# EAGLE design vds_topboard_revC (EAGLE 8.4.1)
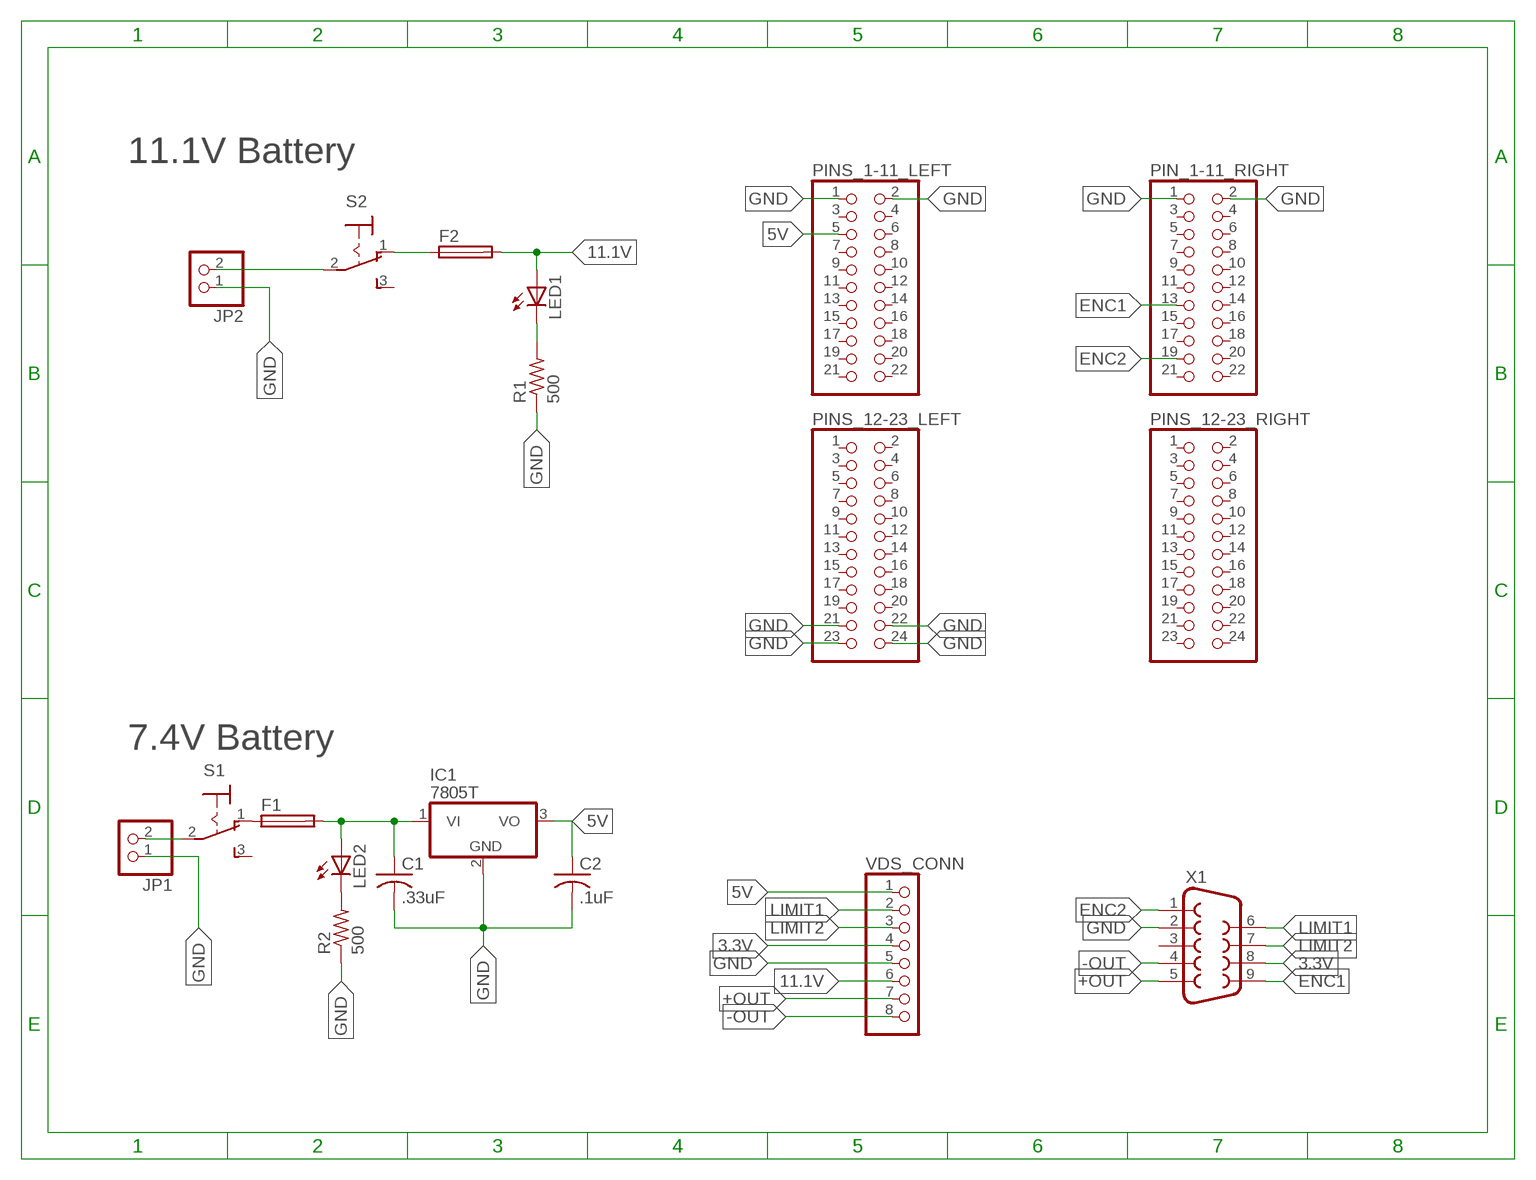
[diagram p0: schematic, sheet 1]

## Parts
C1  .33uF  C-US025-030X050  [C025-030X050]
C2  .1uF  C-US025-030X050  [C025-030X050]
F1  SH22,5  [SH22,5]
F2  SH22,5  [SH22,5]
IC1  7805T  [TO220H]
JP1  PINHD-1X2  [1X02]
JP2  PINHD-1X2  [1X02]
LED1  LED5MM  [LED5MM]
LED2  LED5MM  [LED5MM]
PIN_1-11_RIGHT  PINHD-2X11  [2X11]
PINS_1-11_LEFT  PINHD-2X11  [2X11]
PINS_12-23_LEFT  PINHD-2X12  [2X12]
PINS_12-23_RIGHT  PINHD-2X12  [2X12]
R1  500  R-US_0204/5  [0204/5]
R2  500  R-US_0204/5  [0204/5]
S1  320-916  [320-916]
S2  320-916  [320-916]
VDS_CONN  PINHD-1X8  [1X08]
X1  F09VP  [F09VP]

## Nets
3.3V: VDS_CONN.4 X1.8
5V: C2.1 IC1.3(VO) PINS_1-11_LEFT.5 VDS_CONN.1
7.4VO: C1.1 F1.2 IC1.1(VI) LED2.A
11.1V: F2.2 LED1.A VDS_CONN.6
+OUT: VDS_CONN.7 X1.5
-OUT: VDS_CONN.8 X1.4
ENC1: PIN_1-11_RIGHT.13 X1.9
ENC2: PIN_1-11_RIGHT.19 X1.1
GND: C1.2 C2.2 IC1.2(GND) JP1.1 JP2.1 PIN_1-11_RIGHT.1 PIN_1-11_RIGHT.2 PINS_1-11_LEFT.1 PINS_1-11_LEFT.2 PINS_12-23_LEFT.21 PINS_12-23_LEFT.22 PINS_12-23_LEFT.23 PINS_12-23_LEFT.24 R1.1 R2.1 VDS_CONN.5 X1.2
LIMIT1: VDS_CONN.2 X1.6
LIMIT2: VDS_CONN.3 X1.7
N$1: JP1.2 S1.2(P)
N$2: JP2.2 S2.2(P)
N$4: F2.1 S2.1(O)
N$5: LED1.K(C) R1.2
N$6: LED2.K(C) R2.2
N$7: F1.1 S1.1(O)
Unconnected: PIN_1-11_RIGHT.3 PIN_1-11_RIGHT.4 PIN_1-11_RIGHT.5 PIN_1-11_RIGHT.6 PIN_1-11_RIGHT.7 PIN_1-11_RIGHT.8 PIN_1-11_RIGHT.9 PIN_1-11_RIGHT.10 PIN_1-11_RIGHT.11 PIN_1-11_RIGHT.12 PIN_1-11_RIGHT.14 PIN_1-11_RIGHT.15 PIN_1-11_RIGHT.16 PIN_1-11_RIGHT.17 PIN_1-11_RIGHT.18 PIN_1-11_RIGHT.20 PIN_1-11_RIGHT.21 PIN_1-11_RIGHT.22 PINS_1-11_LEFT.3 PINS_1-11_LEFT.4 PINS_1-11_LEFT.6 PINS_1-11_LEFT.7 PINS_1-11_LEFT.8 PINS_1-11_LEFT.9 PINS_1-11_LEFT.10 PINS_1-11_LEFT.11 PINS_1-11_LEFT.12 PINS_1-11_LEFT.13 PINS_1-11_LEFT.14 PINS_1-11_LEFT.15 PINS_1-11_LEFT.16 PINS_1-11_LEFT.17 PINS_1-11_LEFT.18 PINS_1-11_LEFT.19 PINS_1-11_LEFT.20 PINS_1-11_LEFT.21 PINS_1-11_LEFT.22 PINS_12-23_LEFT.1 PINS_12-23_LEFT.2 PINS_12-23_LEFT.3 PINS_12-23_LEFT.4 PINS_12-23_LEFT.5 PINS_12-23_LEFT.6 PINS_12-23_LEFT.7 PINS_12-23_LEFT.8 PINS_12-23_LEFT.9 PINS_12-23_LEFT.10 PINS_12-23_LEFT.11 PINS_12-23_LEFT.12 PINS_12-23_LEFT.13 PINS_12-23_LEFT.14 PINS_12-23_LEFT.15 PINS_12-23_LEFT.16 PINS_12-23_LEFT.17 PINS_12-23_LEFT.18 PINS_12-23_LEFT.19 PINS_12-23_LEFT.20 PINS_12-23_RIGHT.1 PINS_12-23_RIGHT.2 PINS_12-23_RIGHT.3 PINS_12-23_RIGHT.4 PINS_12-23_RIGHT.5 PINS_12-23_RIGHT.6 PINS_12-23_RIGHT.7 PINS_12-23_RIGHT.8 PINS_12-23_RIGHT.9 PINS_12-23_RIGHT.10 PINS_12-23_RIGHT.11 PINS_12-23_RIGHT.12 PINS_12-23_RIGHT.13 PINS_12-23_RIGHT.14 PINS_12-23_RIGHT.15 PINS_12-23_RIGHT.16 PINS_12-23_RIGHT.17 PINS_12-23_RIGHT.18 PINS_12-23_RIGHT.19 PINS_12-23_RIGHT.20 PINS_12-23_RIGHT.21 PINS_12-23_RIGHT.22 PINS_12-23_RIGHT.23 PINS_12-23_RIGHT.24 S1.3(S) S2.3(S) X1.3

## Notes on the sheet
- 11.1V Battery
- 7.4V Battery

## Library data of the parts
C1 C2 = adafruit:C-US: CAPACITOR, American symbol
F1 F2 = fuse:SH22,5: FUSE HOLDER; MF: SCHURTER; MPN: 0031.8201; OC_FARNELL: 1162740; OC_NEWARK: 96F8317
IC1 = linear:78*: Positive VOLTAGE REGULATOR Source: http://cache.national.com/ds/LM/LM78L05.pdf http://www.fairchildsemi.com/ds/LM/LM7805.pdf
JP1 JP2 = pinhead:PINHD-1X2: PIN HEADER
LED1 LED2 = adafruit:LED: LED
PIN_1-11_RIGHT PINS_1-11_LEFT = pinhead:PINHD-2X11: PIN HEADER
PINS_12-23_LEFT PINS_12-23_RIGHT = pinhead:PINHD-2X12: PIN HEADER
R1 R2 = adafruit:R-US_: RESISTOR, American symbol
S1 S2 = switch:320-916: TOGGLE SWITCH distributor RS Components
VDS_CONN = pinhead:PINHD-1X8: PIN HEADER
X1 = con-subd:F09: SUB-D; OC_FARNELL: unknown; OC_NEWARK: unknown

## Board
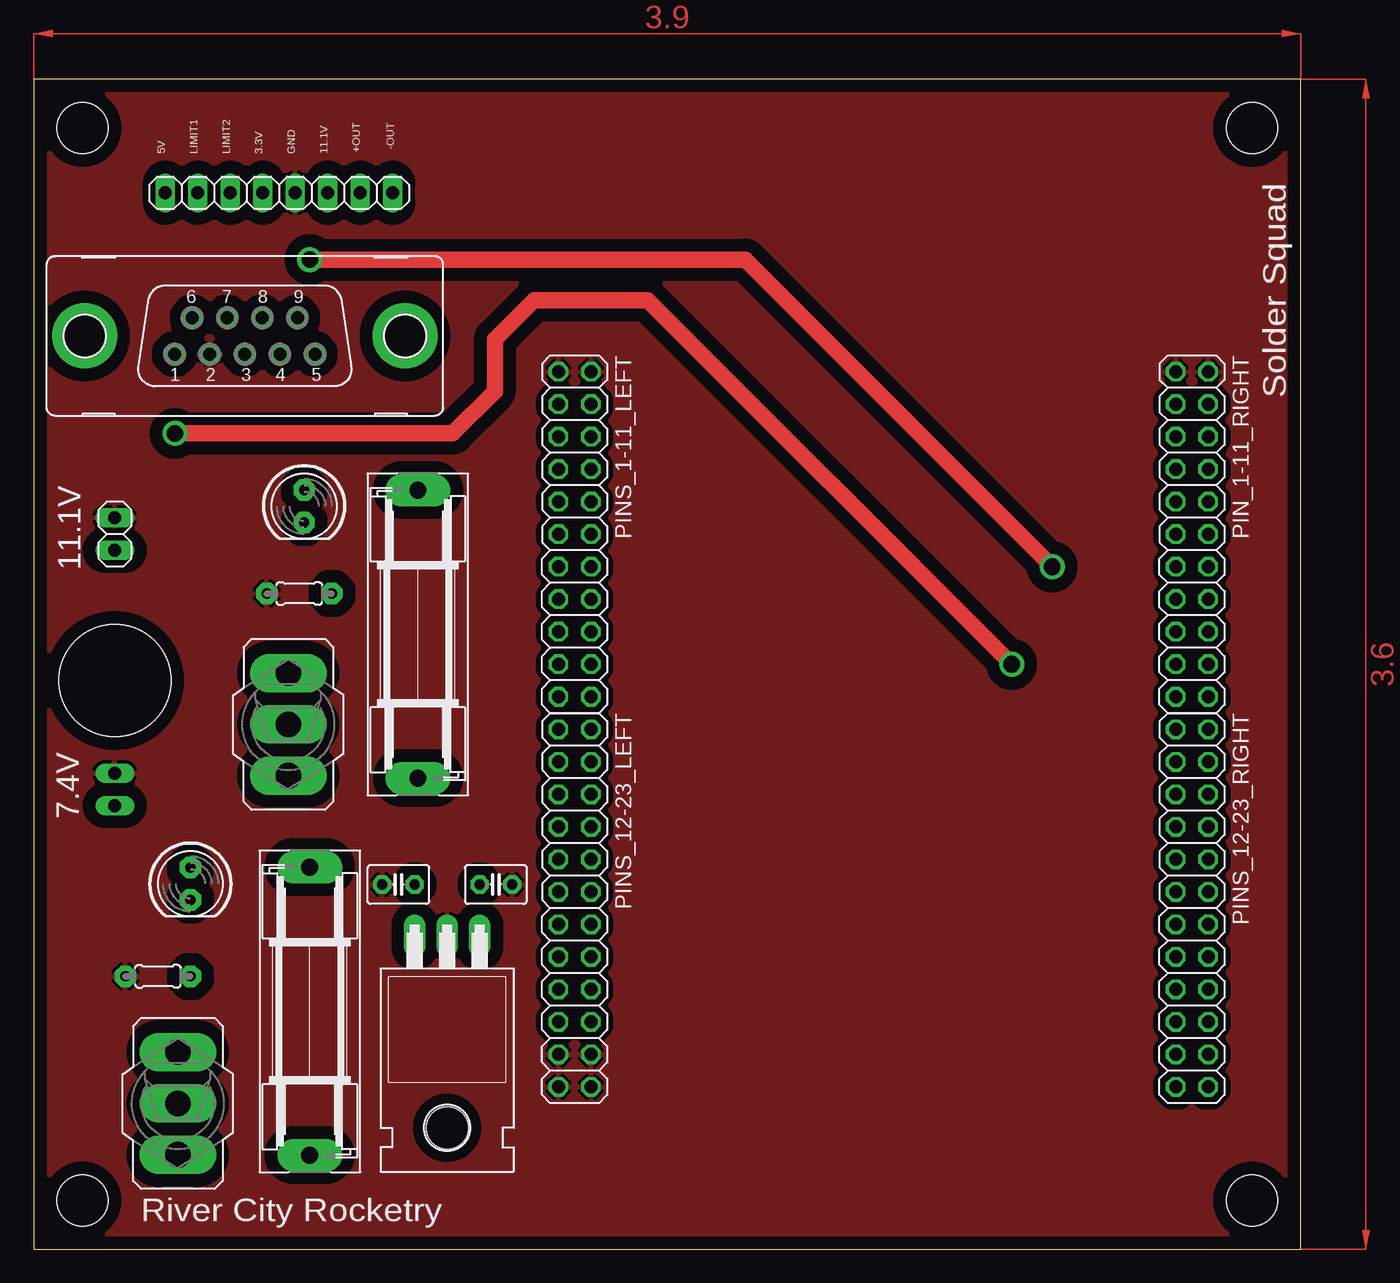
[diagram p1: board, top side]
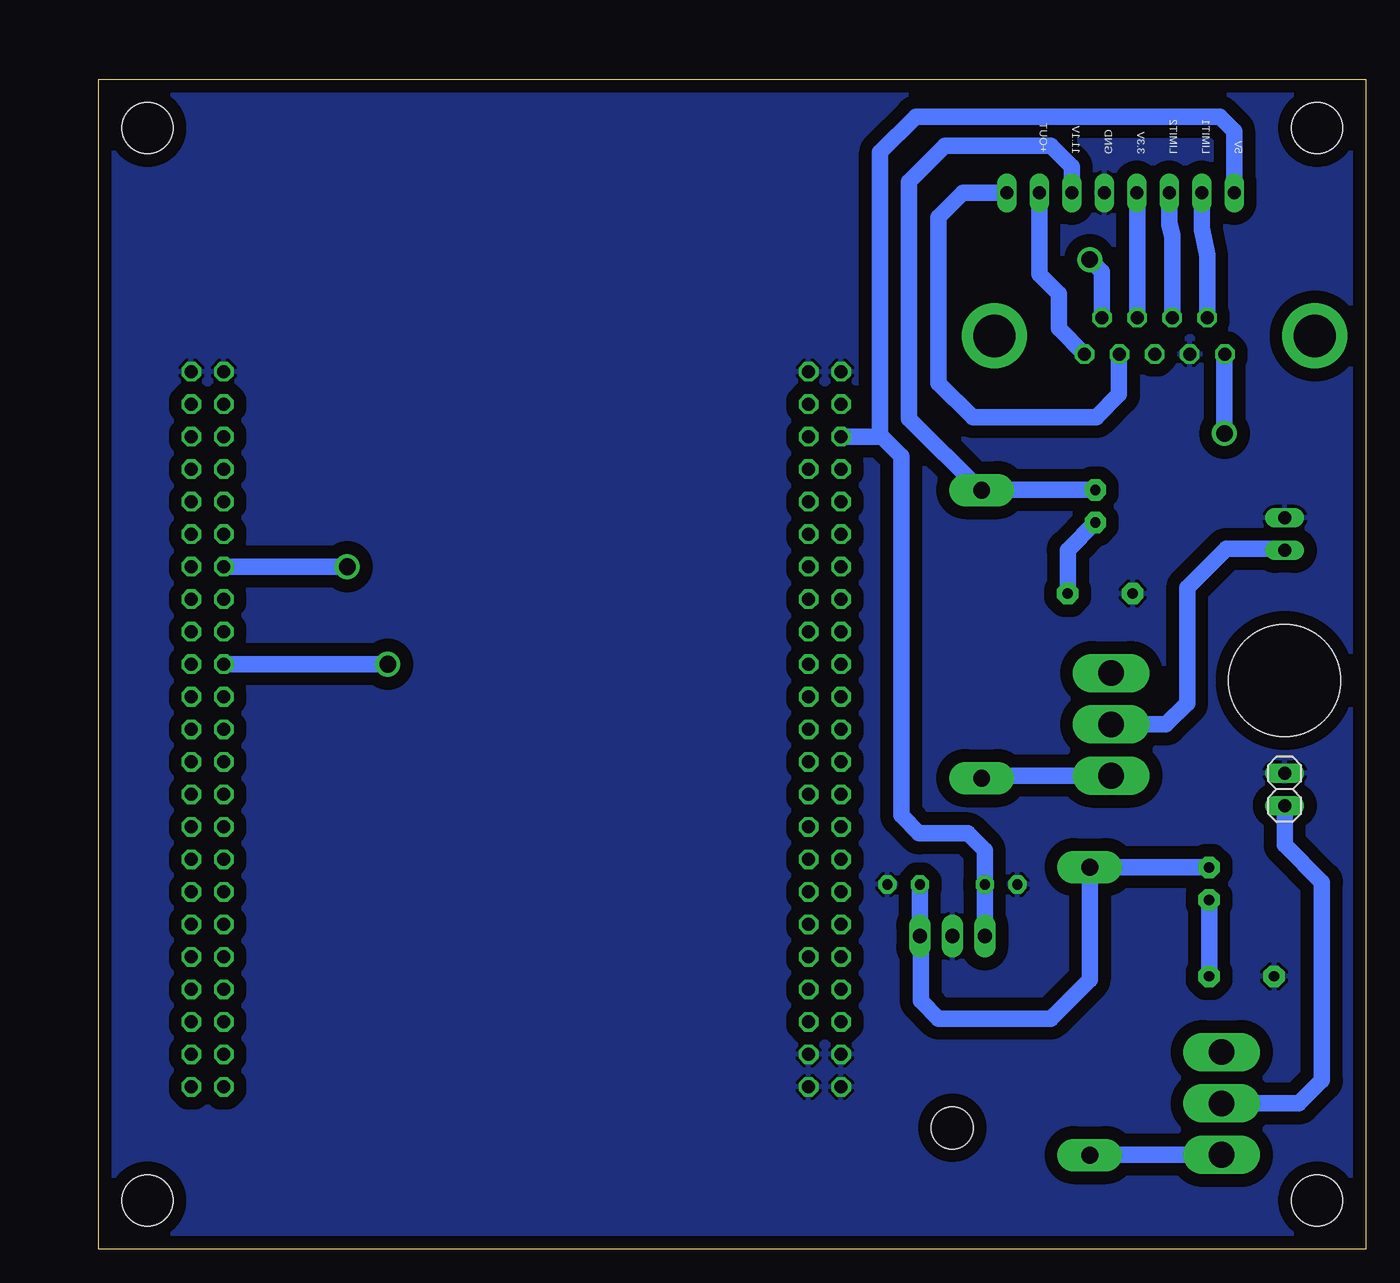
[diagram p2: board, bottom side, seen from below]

Size 99.06 x 91.44 mm. Coordinates in mm from the lower left corner, seen from the top.
Outline: 0,0 99.06,0 99.06,91.44 0,91.44 0,0
Copper layers (1*16): Top 0.035mm / dielectric 1.5mm / Bottom 0.035mm
Design rules "default *": minimum track width 10mil, minimum drill 24mil, track to track 1mm, track to pad 1mm, pad to pad 1mm, via to via 1mm, smd to smd 1mm, copper to edge 40mil, drill to drill 8mil, minimum pad ring 10mil, minimum via ring 8mil, stop-mask expansion 4mil, vias tented up to drill 0mil, thermal gap 10mil
Holes 4 mm at 3.81,3.81 3.81,87.63 95.25,87.63 95.25,3.81
Holes 8.76 mm at 6.35,44.45

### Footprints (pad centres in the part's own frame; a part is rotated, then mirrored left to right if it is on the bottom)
C025-030X050 = drill 0.813 pad 1.422 octagon: 1 -1.27,0; 2 1.27,0
SH22,5 = drill 1.321 pad 2.54 long: 1 -11.252,0; 2 11.252,0
TO220H = drill 1.118 long: 1 -2.54,-10.16; 2 0,-10.16; 3 2.54,-10.16 | hole 3.302: 0,4.826
1X02 = drill 1.016 long: 1 -1.27,0; 2 1.27,0
LED5MM = drill 0.813 pad 1.676 octagon: A -1.27,0; K 1.27,0
2X11 = drill 1.016 octagon: 1 -12.7,-1.27; 2 -12.7,1.27; 3 -10.16,-1.27; 4 -10.16,1.27; 5 -7.62,-1.27; 6 -7.62,1.27; 7 -5.08,-1.27; 8 -5.08,1.27; 9 -2.54,-1.27; 10 -2.54,1.27; 11 0,-1.27; 12 0,1.27; 13 2.54,-1.27; 14 2.54,1.27; 15 5.08,-1.27; 16 5.08,1.27; 17 7.62,-1.27; 18 7.62,1.27; 19 10.16,-1.27; 20 10.16,1.27; 21 12.7,-1.27; 22 12.7,1.27
2X12 = drill 1.016 octagon: 1 -13.97,-1.27; 2 -13.97,1.27; 3 -11.43,-1.27; 4 -11.43,1.27; 5 -8.89,-1.27; 6 -8.89,1.27; 7 -6.35,-1.27; 8 -6.35,1.27; 9 -3.81,-1.27; 10 -3.81,1.27; 11 -1.27,-1.27; 12 -1.27,1.27; 13 1.27,-1.27; 14 1.27,1.27; 15 3.81,-1.27; 16 3.81,1.27; 17 6.35,-1.27; 18 6.35,1.27; 19 8.89,-1.27; 20 8.89,1.27; 21 11.43,-1.27; 22 11.43,1.27; 23 13.97,-1.27; 24 13.97,1.27
0204/5 = drill 0.813 pad 1.676 octagon: 1 -2.54,0; 2 2.54,0
320-916 = drill 2.007 long: 1 0,4.013; 2 0,0; 3 0,-4.013
1X08 = drill 1.016 long: 1 -8.89,0; 2 -6.35,0; 3 -3.81,0; 4 -1.27,0; 5 1.27,0; 6 3.81,0; 7 6.35,0; 8 8.89,0
F09VP = drill 1.016 octagon: 1 5.486,1.422; 2 2.743,1.422; 3 0,1.422; 4 -2.743,1.422; 5 -5.486,1.422; 6 4.115,-1.422; 7 1.372,-1.422; 8 -1.372,-1.422; 9 -4.115,-1.422 | drill 3.302 pad 5.08: G1 -12.522,0; G2 12.522,0

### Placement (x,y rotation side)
C1  36.13,28.51 0 top
C2  28.51,28.51 180 top
F1  21.59,18.61 90 top
F2  30.04,48.07 90 top
IC1  32.32,14.32 180 top
JP1  6.35,35.94 270 bottom
JP2  6.35,55.88 270 top
LED1  21.15,58.07 270 top
LED2  12.26,28.57 270 top
PIN_1-11_RIGHT  90.55,55.88 270 top
PINS_1-11_LEFT  42.29,55.88 270 top
PINS_12-23_LEFT  42.29,26.67 270 top
PINS_12-23_RIGHT  90.55,26.67 270 top
R1  20.76,51.24 0 top
R2  9.72,21.34 0 top
S1  11.27,11.4 180 top
S2  19.91,41.02 180 top
VDS_CONN  19.18,82.55 0 top
X1  16.51,71.37 180 top

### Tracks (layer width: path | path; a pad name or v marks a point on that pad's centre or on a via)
3.3V
  Bottom 1.27: X1.8 17.88,82.53 VDS_CONN.4
5V
  Bottom 1.27: IC1.3 C2.1 29.78,31.18 31.11,32.51 34.92,32.51 36.32,33.91 36.32,61.98 37.85,63.5 | 37.85,63.5 PINS_1-11_LEFT.5 | VDS_CONN.1 10.29,87.38 11.43,88.52 35.18,88.52 37.97,85.72 37.97,63.63 37.85,63.5
7.4VO  (via drill 0.35)
  Bottom 1.27: C1.1 IC1.1 v34.8,24.42 34.8,19.43 33.4,18.03 24.64,18.03 21.59,21.08 F1.2 21.58,29.84 LED2.A
11.1V
  Bottom 1.27: LED1.A 30.02,59.34 F2.2 30.11,59.32 35.7,64.91 35.7,83.42 32.89,86.23 24.64,86.23 22.99,84.58 VDS_CONN.6
+OUT
  Bottom 1.27: X1.5 24,71.96 24,74.68 25.53,76.2 VDS_CONN.7
-OUT
  Bottom 1.27: X1.4 19.3,69.9 19.3,66.8 21.08,65.02 30.73,65.02 33.4,67.69 33.4,80.64 31.5,82.55 VDS_CONN.8
ENC1  (via drill 1.3 pad 1.95)
  Top 1.27: v21.59,77.34 55.63,77.34 v79.63,53.34
  Bottom 1.27: X1.9 20.62,76.38 v21.59,77.34 | v79.63,53.34 PIN_1-11_RIGHT.13
ENC2  (via drill 1.3 pad 1.95)
  Top 1.27: v11.05,63.75 32.77,63.75 36.07,67.06 36.07,71.12 39.12,74.17 48.01,74.17 v76.45,45.72
  Bottom 1.27: 10.95,69.95 X1.1 11.05,69.93 v11.05,63.75 | v76.45,45.72 PIN_1-11_RIGHT.19
GND
  pour Top: 0,91.44 0,0 99.06,0 99.06,91.44
  pour Bottom: 0,91.44 0,0 99.06,0 99.06,91.44
LIMIT1
  Bottom 1.27: X1.6 12.39,77.67 12.83,79.76 VDS_CONN.2
LIMIT2
  Bottom 1.27: X1.7 15.14,79.15 15.37,80.14 VDS_CONN.3
N$1
  Bottom 1.27: S1.2 5.24,11.4 3.43,13.21 3.43,28.7 6.35,31.62 JP1.2
N$2
  Bottom 1.27: S2.2 15.62,41.02 13.97,42.67 13.97,51.69 10.92,54.74 6.48,54.74 JP2.2
N$4
  Bottom 1.27: S2.1 29.84,37.01 F2.1
N$5
  Bottom 1.27: LED1.K 23.3,54.64 R1.2
N$6
  Bottom 1.27: R2.2 LED2.K
N$7
  Bottom 1.27: S1.1 21.56,7.38 F1.1
(copper drawn outside any net)
  shapes: Top area x2

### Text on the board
tPlace: 5V | LIMIT1 | LIMIT2 | 3.3V | GND | 11.1V | +OUT | -OUT | Solder Squad | 11.1V | 7.4V | River City Rocketry
bPlace: 5V | LIMIT1 | LIMIT2 | 3.3V | GND | 11.1V | +OUT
